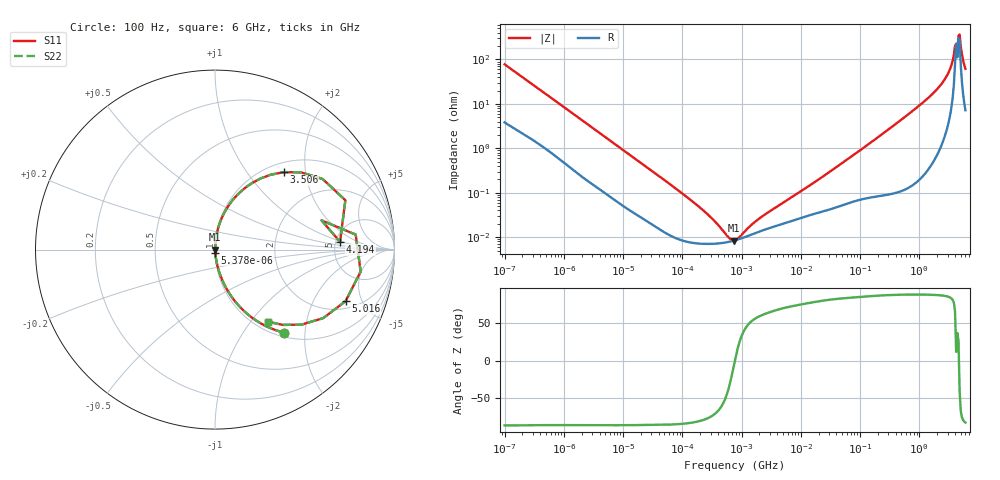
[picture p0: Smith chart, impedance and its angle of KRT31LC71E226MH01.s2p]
!Murata Part Number: KRT31LC71E226MH01
!These Parameters are Measured in Series Mode Connection
!Data Generated on Jan 08, 2026
!  o--ll--o
!Port1  Port2
!  o------o
!Operation Temp=25[degC], DC Bias Voltage=0[V]
!Freq. Start=100[Hz] Stop=6[GHz] 401[Steps]
# Hz S RI R 50
!Freq.(Hz) S11(Real) S11(Imag) S21(Real) S21(Imag) S12(Real) S12(Imag) S22(Real) S22(Imag)
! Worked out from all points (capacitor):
!   401 points, 100 Hz to 6 GHz, reference 50 ohm
!   read as one part in series: C = 20.2 uF near 109 Hz
!   lowest |Z| = 8.41 mohm at 740.7 kHz (marker M1)
!   series resonance near 771.4 kHz, so ESL is about 2.1 nH
!   S11 on the Smith chart (normalised r, x): 100 Hz: 1.08, -1.56; 5.378 kHz: 1.00, -0.03; 3.506 GHz: 1.18, +1.52; 4.194 GHz: 5.46, +0.92; 5.016 GHz: 2.48, -3.67; 6 GHz: 1.14, -1.23
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100  0.3835 -0.4623  0.6165 0.4623  0.6165 0.4623  0.3835 -0.4623
306  0.0775 -0.2403  0.9225 0.2403  0.9225 0.2403  0.0775 -0.2403
2008  0.00416 -0.043  0.9958 0.043  0.9958 0.043  0.00416 -0.043
5378  0.00118 -0.0167  0.9988 0.0167  0.9988 0.0167  0.00118 -0.0167
40335  0.000159 -0.00237  0.9998 0.00237  0.9998 0.00237  0.000159 -0.00237
221108  7.1e-05 -0.000404  0.9999 0.000404  0.9999 0.000404  7.1e-05 -0.000404
566185  7.7e-05 -7.71e-05  0.9999 7.71e-05  0.9999 7.71e-05  7.7e-05 -7.71e-05
740679  8.35e-05 -9.7e-06  0.9999 9.7e-06  0.9999 9.7e-06  8.35e-05 -9.7e-06
774597  8.49e-05 1e-06  0.9999 -1e-06  0.9999 -1e-06  8.49e-05 1e-06
968953  9.32e-05 5.38e-05  0.9999 -5.38e-05  0.9999 -5.38e-05  9.32e-05 5.38e-05
2074311  0.000136 0.000238  0.9999 -0.000238  0.9999 -0.000238  0.000136 0.000238
1.555665e7  0.000327 0.00155  0.9997 -0.00155  0.9997 -0.00155  0.000327 0.00155
3.124326e8  0.00168 0.0275  0.9983 -0.0275  0.9983 -0.0275  0.00168 0.0275
1.000774e9  0.0103 0.0907  0.9897 -0.0907  0.9897 -0.0907  0.0103 0.0907
2.048624e9  0.0537 0.2091  0.9463 -0.2091  0.9463 -0.2091  0.0537 0.2091
2.931063e9  0.1732 0.3482  0.8268 -0.3482  0.8268 -0.3482  0.1732 0.3482
3.505958e9  0.383 0.4317  0.617 -0.4317  0.617 -0.4317  0.383 0.4317
4.193612e9  0.6967 0.0433  0.3033 -0.0433  0.3033 -0.0433  0.6967 0.0433
4.586474e9  0.7839 0.0836  0.2161 -0.0836  0.2161 -0.0836  0.7839 0.0836
5.016141e9  0.7277 -0.2871  0.2723 0.2871  0.2723 0.2871  0.7277 -0.2871
5.486059e9  0.481 -0.4184  0.519 0.4184  0.519 0.4184  0.481 -0.4184
6e9  0.2968 -0.4019  0.7032 0.4019  0.7032 0.4019  0.2968 -0.4019
